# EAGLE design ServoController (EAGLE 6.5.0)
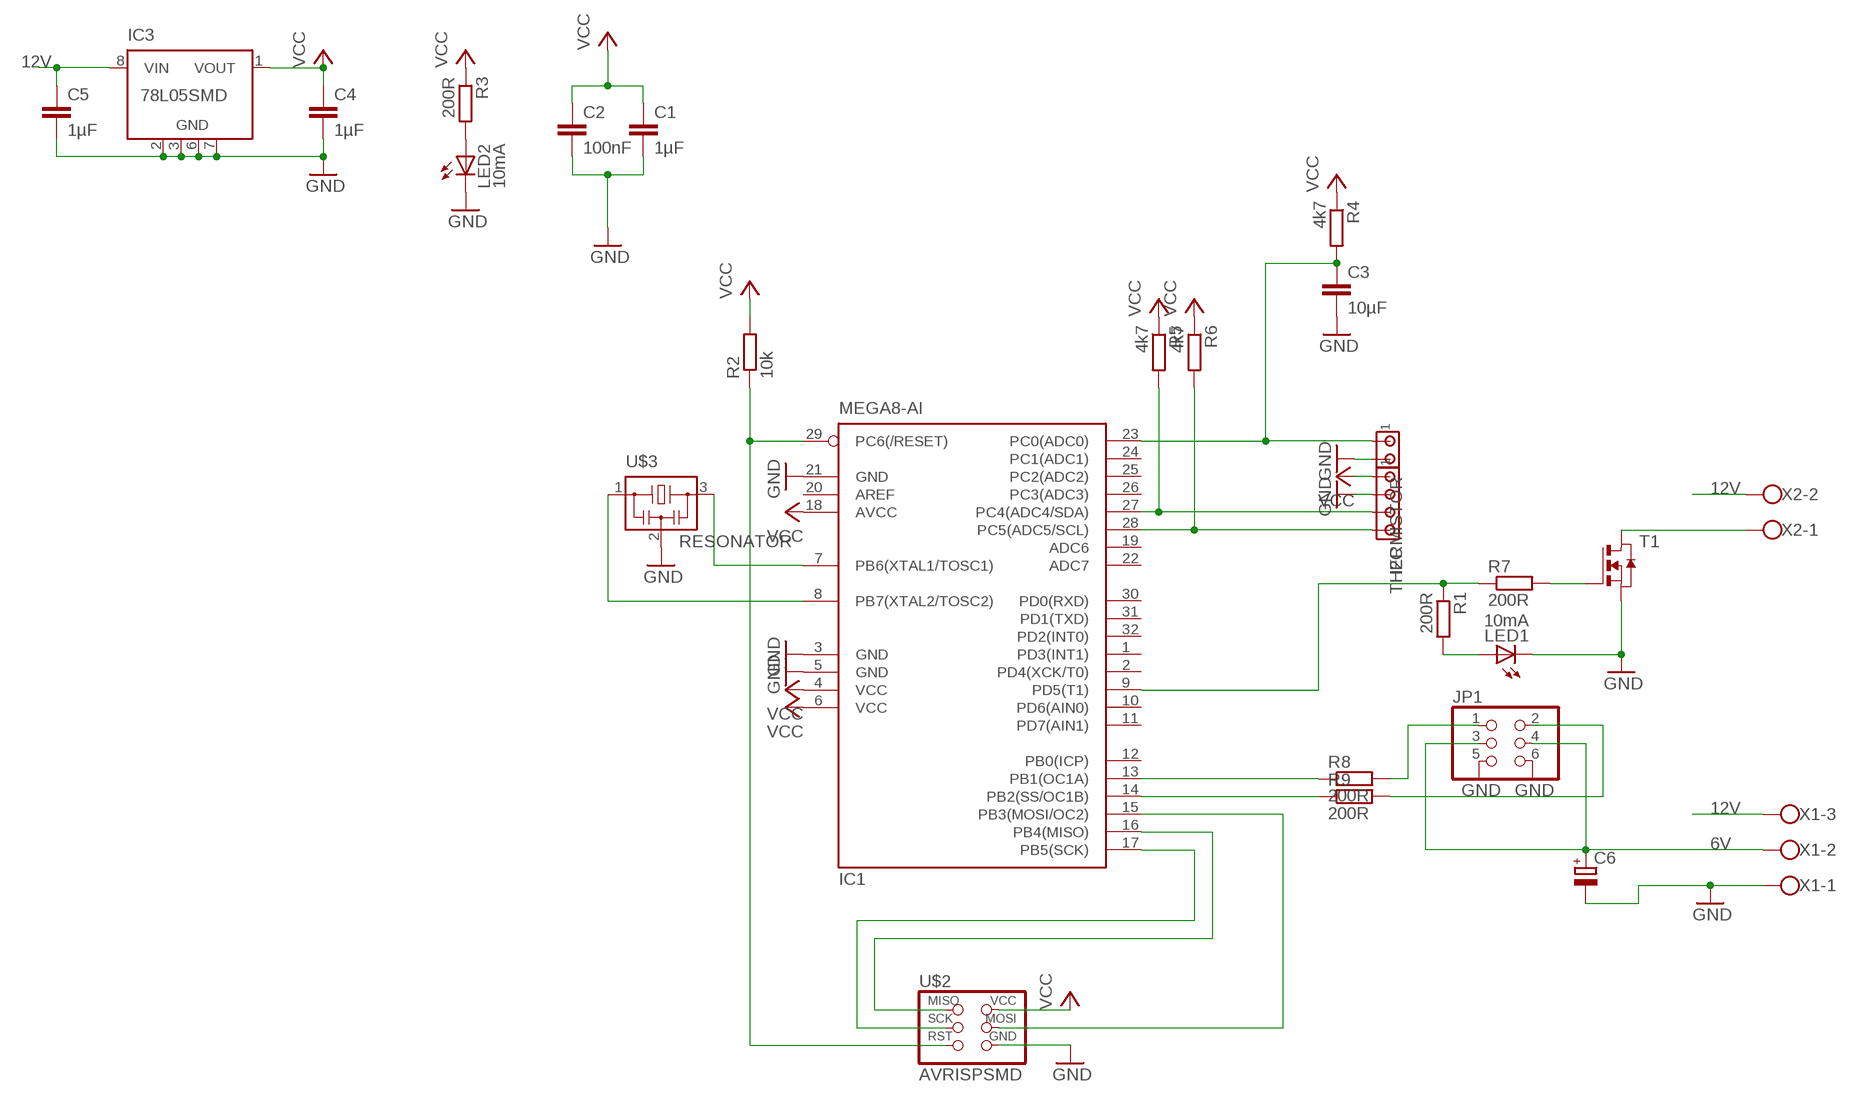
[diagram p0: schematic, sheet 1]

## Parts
C1  1µF  C-EUC1206  [C1206]
C2  100nF  C-EUC1206  [C1206]
C3  10µF  C-EUC1206  [C1206]
C4  1µF  C-EUC1206  [C1206]
C5  1µF  C-EUC1206  [C1206]
C6  CPOL-EUE10-25  [EB25D]
I2C  MTA04-100  [10X04MTA]
IC1  MEGA8-AI  [TQFP32-08]
IC3  78L05SMD  [SO08]
JP1  PINHD-2X3-SMD  [2X03SMD]
LED1  10mA  LEDCHIPLED_1206  [CHIPLED_1206]
LED2  10mA  LEDCHIPLED_1206  [CHIPLED_1206]
R1  200R  R-EU_R1206  [R1206]
R2  10k  R-EU_R1206  [R1206]
R3  200R  R-EU_R1206  [R1206]
R4  4k7  R-EU_R1206  [R1206]
R5  4k7  R-EU_R1206  [R1206]
R6  4k7  R-EU_R1206  [R1206]
R7  200R  R-EU_R1206  [R1206]
R8  200R  R-EU_R1206  [R1206]
R9  200R  R-EU_R1206  [R1206]
T1  NMOSSOT23-6  [SOT23-6]
THERMISTOR  MTA02-100  [10X02MTA]
U$2  AVRISPSMD  [2X03SMD]
U$3  RESONATOR  [EFOBM]
X1  W237-103  [W237-103]
X2  W237-102  [W237-102]

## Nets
6V: C6.+ JP1.3 JP1.4 X1.2
12V: C5.1 IC3.8(VIN) X1.3 X2.2
GND: C1.2 C2.2 C3.2 C4.2 C5.2 C6.- I2C.2 IC1.3(GND) IC1.5(GND) IC1.21(GND) IC3.2(GND) IC3.3(GND) IC3.6(GND) IC3.7(GND) JP1.5 JP1.6 LED1.C LED2.C T1.4(S) THERMISTOR.2 U$2.6(GND) U$3.2 X1.1
N$1: IC1.13(PB1(OC1A)) R8.1
N$2: IC1.29(PC6(/RESET)) R2.1 U$2.5(RST)
N$3: JP1.2 R9.2
N$4: IC1.15(PB3(MOSI/OC2)) U$2.4(MOSI)
N$5: IC1.16(PB4(MISO)) U$2.1(MISO)
N$6: IC1.8(PB7(XTAL2/TOSC2)) U$3.1
N$7: IC1.7(PB6(XTAL1/TOSC1)) U$3.3
N$8: IC1.17(PB5(SCK)) U$2.3(SCK)
N$9: IC1.9(PD5(T1)) R1.1 R7.1
N$10: LED1.A R1.2
N$11: T1.1(D) T1.2(D) T1.5(D) T1.6(D) X2.1
N$12: LED2.A R3.2
N$13: I2C.3 IC1.27(PC4(ADC4/SDA)) R5.2
N$14: I2C.4 IC1.28(PC5(ADC5/SCL)) R6.2
N$15: C3.1 IC1.23(PC0(ADC0)) R4.2 THERMISTOR.1
N$16: R7.2 T1.3(G)
N$17: IC1.14(PB2(SS/OC1B)) R9.1
N$18: JP1.1 R8.2
VCC: C1.1 C2.1 C4.1 I2C.1 IC1.4(VCC) IC1.6(VCC) IC1.18(AVCC) IC3.1(VOUT) R2.2 R3.1 R4.1 R5.1 R6.1 U$2.2(VCC)
Unconnected: IC1.1(PD3(INT1)) IC1.2(PD4(XCK/T0)) IC1.10(PD6(AIN0)) IC1.11(PD7(AIN1)) IC1.12(PB0(ICP)) IC1.19(ADC6) IC1.20(AREF) IC1.22(ADC7) IC1.24(PC1(ADC1)) IC1.25(PC2(ADC2)) IC1.26(PC3(ADC3)) IC1.30(PD0(RXD)) IC1.31(PD1(TXD)) IC1.32(PD2(INT0)) IC3.4(NC) IC3.5(NC)

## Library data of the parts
C1-C5 = resistor:C-EU: CAPACITOR, European symbol
C6 = rcl:CPOL-EU: POLARIZED CAPACITOR, European symbol
I2C = con-amp:MTA04-100: AMP connector
IC1 = atmel:MEGA8: MICROCONTROLLER 8 Kbytes FLASH, 1 kbytes SRAM, 512 bytes EEPROM, USART, 6-channel 10 bit ADC, 2-channel 8 bit ADC Pin compatible with Atmega48, ATMega88, ATMega168 Source: avr.lbr; MPN: ATMEGA8-16AU; OC_FARNELL: 9171371; OC_NEWARK: 73M8863
IC3 = linear:78L*SMD: Positive VOLTAGE REGULATOR
JP1 = fab:PINHD-2X3-SMD: PIN HEADER
LED1 LED2 = led:LED: LED
R1-R9 = resistor:R-EU_: RESISTOR, European symbol
T1 = zetex:NMOSSOT23-6: MOS FET; OC_FARNELL: unknown; OC_NEWARK: unknown
THERMISTOR = con-amp:MTA02-100: AMP connector
U$2 = fab:AVRISP
U$3 = fab:RESONATOR
X1 = con-wago-500:W237-103: WAGO SCREW CLAMP; MPN: 237-103; OC_FARNELL: unknown; OC_NEWARK: 18M7116
X2 = con-wago-500:W237-102: WAGO SCREW CLAMP; MPN: 237-102; OC_FARNELL: unknown; OC_NEWARK: 70K9898

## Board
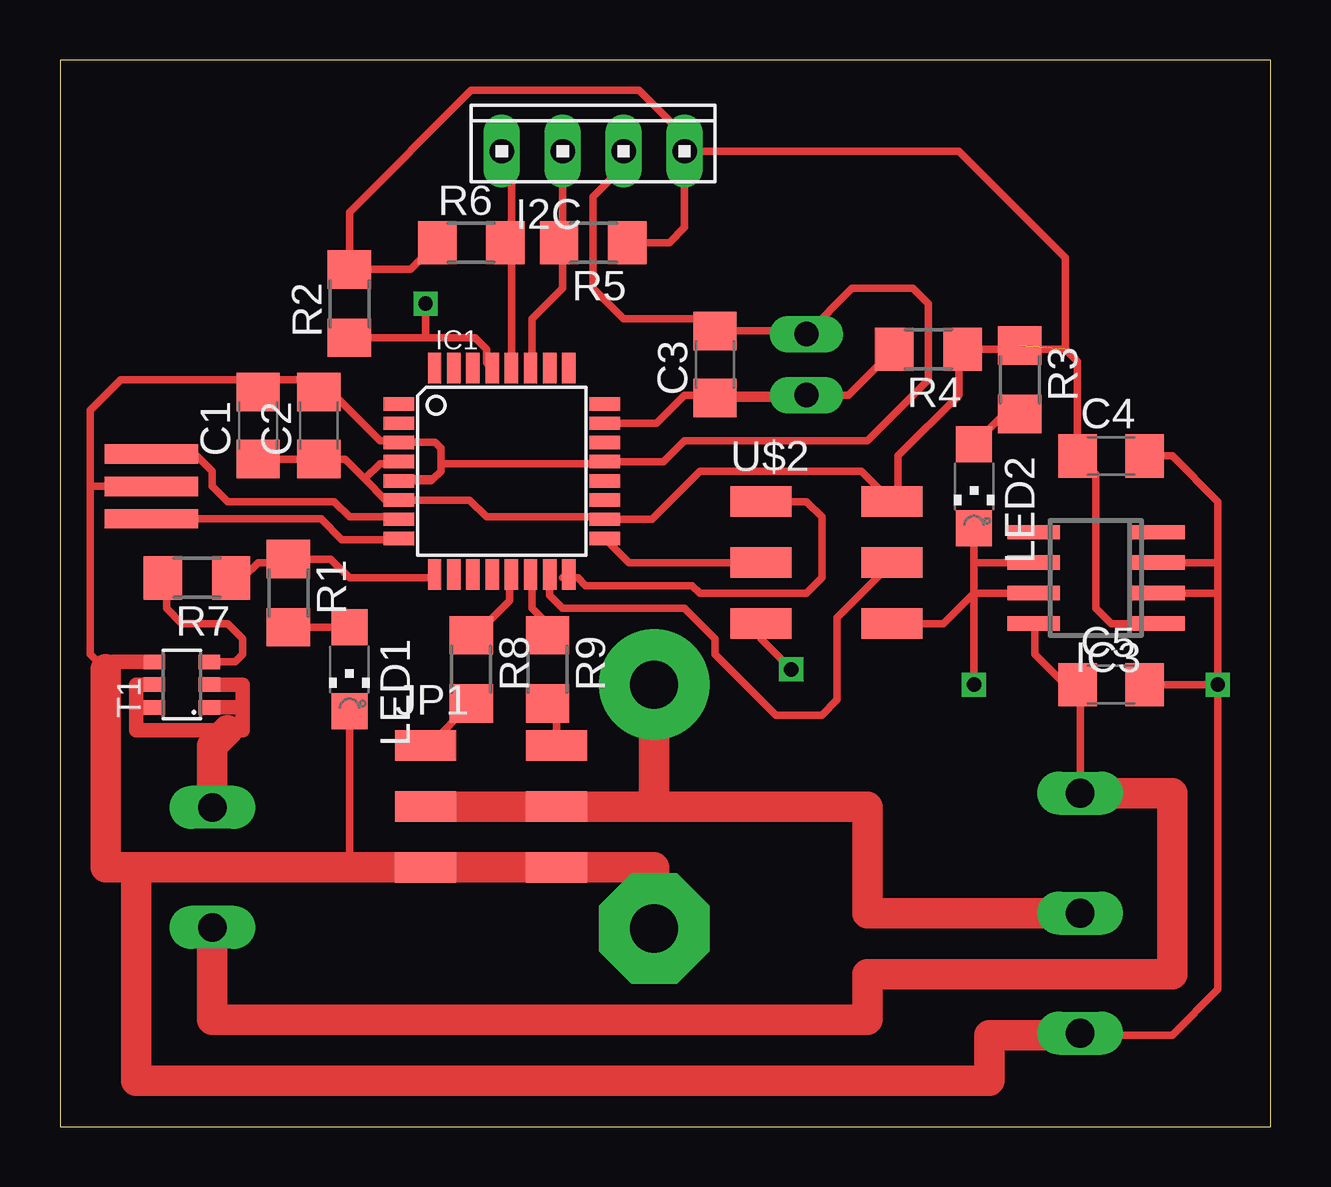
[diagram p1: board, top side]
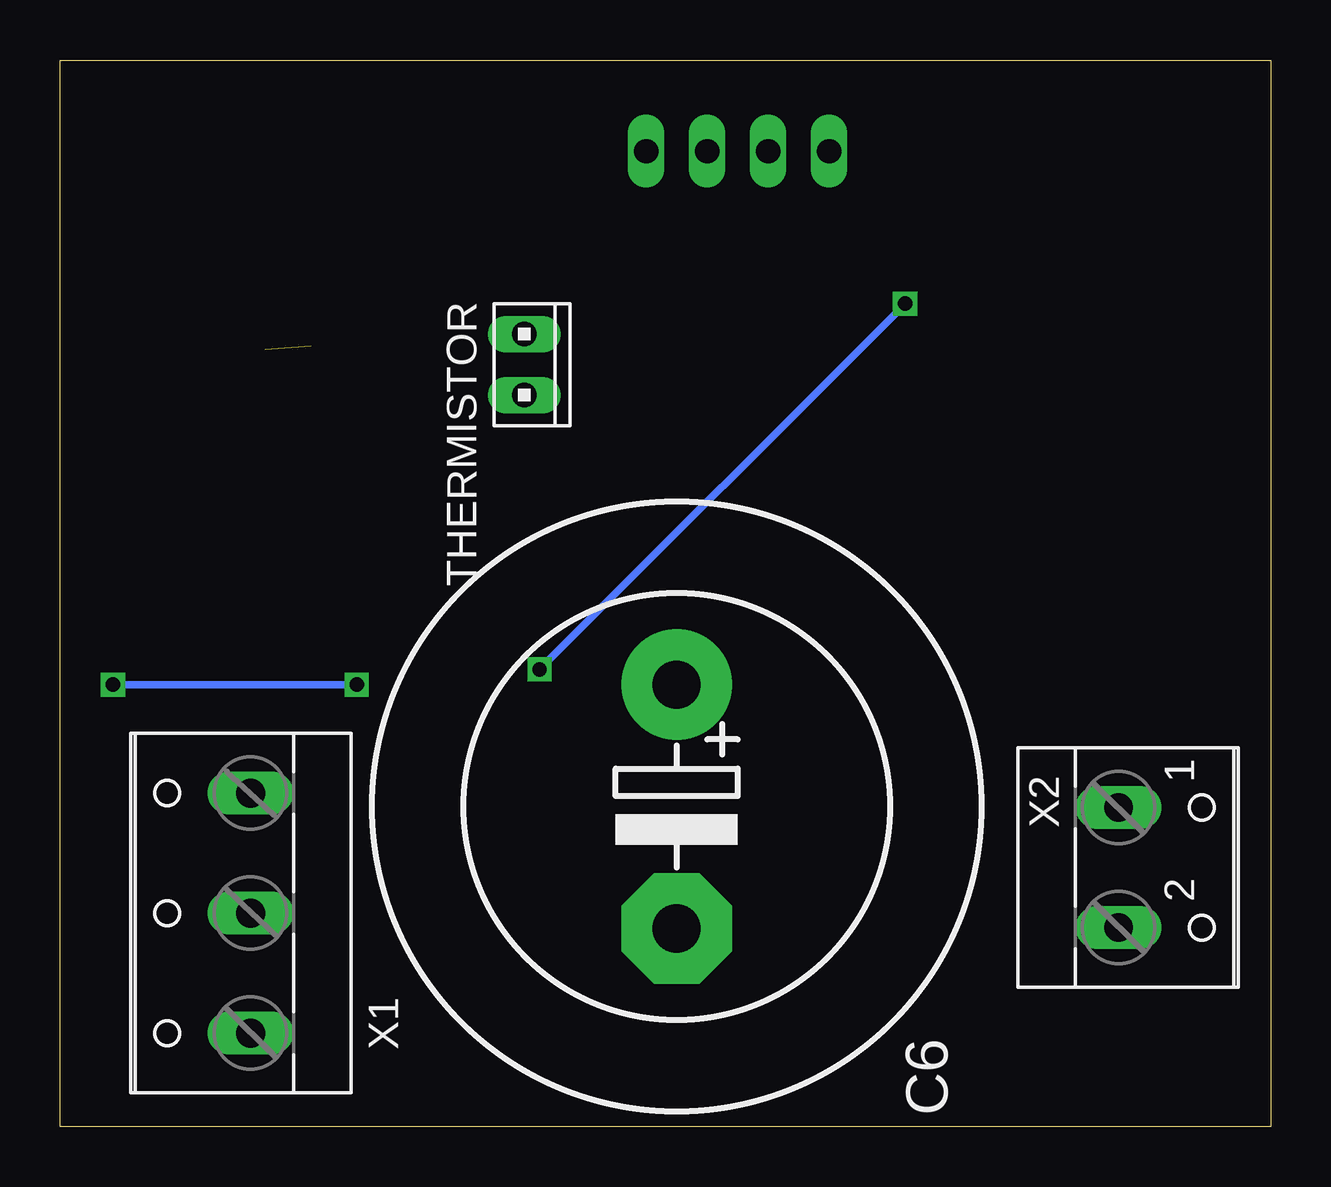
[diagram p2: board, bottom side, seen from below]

Size 50.47 x 44.44 mm. Coordinates in mm from the lower left corner, seen from the top.
Outline: 0,0 50.47,0 50.47,44.44 0,44.44 0,0
Copper layers (1*16): Top 0.035mm / dielectric 1.5mm / Bottom 0.035mm
Design rules "fab": minimum track width 0.3mm, minimum drill 32mil, track to track 0.315mm, track to pad 0.315mm, pad to pad 0.315mm, via to via 0.315mm, smd to smd 0.315mm, copper to edge 40mil, drill to drill 16mil, minimum pad ring 10mil, minimum via ring 8mil, stop-mask expansion 4mil, vias tented up to drill 0mil, thermal gap 10mil

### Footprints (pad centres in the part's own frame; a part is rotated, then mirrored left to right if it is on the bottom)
C1206 = smd 1.6 x 1.8: 1 -1.4,0; 2 1.4,0
EB25D = drill 2.007 pad 4.597: + -5.08,0 | drill 2.007 pad 4.597 octagon: - 5.08,0
10X04MTA = drill 1.016 long: 1 3.81,0; 2 1.27,0; 3 -1.27,0; 4 -3.81,0
TQFP32-08 = smd 1.27 x 0.559: 1 -4.293,2.8; 2 -4.293,2; 3 -4.293,1.2; 4 -4.293,0.4; 5 -4.293,-0.4; 6 -4.293,-1.2; 7 -4.293,-2; 8 -4.293,-2.8; 17 4.293,-2.8; 18 4.293,-2; 19 4.293,-1.2; 20 4.293,-0.4; 21 4.293,0.4; 22 4.293,1.2; 23 4.293,2; 24 4.293,2.8 | smd 0.559 x 1.27: 9 -2.8,-4.293; 10 -2,-4.293; 11 -1.2,-4.293; 12 -0.4,-4.293; 13 0.4,-4.293; 14 1.2,-4.293; 15 2,-4.293; 16 2.8,-4.293; 25 2.8,4.293; 26 2,4.293; 27 1.2,4.293; 28 0.4,4.293; 29 -0.4,4.293; 30 -1.2,4.293; 31 -2,4.293; 32 -2.8,4.293
SO08 = smd 0.6 x 2.2: 1 -1.905,-2.6; 2 -0.635,-2.6; 3 0.635,-2.6; 4 1.905,-2.6; 5 1.905,2.6; 6 0.635,2.6; 7 -0.635,2.6; 8 -1.905,2.6
2X03SMD = smd 2.54 x 1.27: 1 -2.54,2.54; 2 2.92,2.54; 3 -2.54,0; 4 2.92,0; 5 -2.54,-2.54; 6 2.92,-2.54
CHIPLED_1206 = smd 1.5 x 1.5: A 0,-1.75; C 0,1.75
R1206 = smd 1.6 x 1.803: 1 -1.422,0; 2 1.422,0
SOT23-6 = smd 0.6 x 0.9: 1 -0.95,-1.15; 2 0,-1.15; 3 0.95,-1.15; 4 0.95,1.15; 5 0,1.15; 6 -0.95,1.15
10X02MTA = drill 1.016 long: 1 1.27,0; 2 -1.27,0
EFOBM = smd 0.8 x 3.9: 1 -1.35,0; 2 0,0; 3 1.35,0
W237-103 = drill 1.194 long: 1 -5,-1.29; 2 0,-1.29; 3 5,-1.29
W237-102 = drill 1.194 long: 1 -2.5,-1.27; 2 2.5,-1.27

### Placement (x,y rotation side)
C1  8.26,29.21 90 top
C2  10.79,29.21 90 top
C3  27.3,31.75 90 top
C4  43.81,27.94 0 top
C5  43.81,18.41 0 top
C6  24.77,13.34 270 bottom
I2C  22.23,40.64 0 top
IC1  18.41,27.3 0 top
IC3  43.18,22.86 90 top
JP1  17.78,13.34 0 top
LED1  12.06,19.05 180 top
LED2  38.1,26.67 180 top
R1  9.53,22.23 270 top
R2  12.06,34.29 90 top
R3  40.01,31.11 270 top
R4  36.2,32.38 180 top
R5  22.23,36.83 180 top
R6  17.14,36.83 0 top
R7  5.71,22.86 180 top
R8  17.14,19.05 270 top
R9  20.32,19.05 270 top
T1  5.08,18.41 90 top
THERMISTOR  31.11,31.75 270 bottom
U$2  31.75,23.5 0 top
U$3  3.81,26.67 90 top
X1  43.81,8.89 90 bottom
X2  5.08,10.79 270 bottom

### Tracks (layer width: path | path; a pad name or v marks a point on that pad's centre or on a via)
6V
  Top 1.27: JP1.3 JP1.4 24.77,13.34 | 24.77,13.34 33.66,13.34 33.66,8.89 X1.2 | 24.77,13.34 C6.+
12V
  Top 0.305: X1.3 42.52,18.3 C5.1 41.91,18.41 40.64,19.68 40.64,20.89 IC3.8
  Top 1.27: X1.3 46.35,13.89 46.35,6.35 33.66,6.35 33.66,4.45 6.35,4.45 X2.2
GND  (via drill 0.6)
  Top 0.305: 8.26,31.11 10.79,31.11 | 10.79,31.11 13.34,28.57 14.05,28.57 IC1.3 15.63,28.5 15.88,28.26 15.88,27.62 | 15.56,26.99 15.88,27.3 15.88,27.62 | 15.56,26.99 14.21,26.99 IC1.5 15.47,26.91 15.56,26.99 | 15.88,27.62 22.62,27.62 IC1.21 25.16,27.7 26.04,28.57 33.66,28.57 36.2,31.11 36.2,34.29 35.56,34.92 33.02,34.92 THERMISTOR.2 30.98,33.15 C3.2 26.8,33.66 23.5,33.66 22.23,34.92 22.23,38.73 23.5,40.01 I2C.2 23.5,41.91 | LED1.C 12.06,10.79 | v48.26,18.41 48.26,5.71 46.35,3.81 42.6,3.81 X1.1 | 46.35,18.41 C5.2 v48.26,18.41 | 38.1,22.23 36.83,20.95 U$2.6 | IC3.7 38.1,22.23 | IC3.3 48.26,23.5 | 48.26,23.5 48.26,22.23 | 48.26,22.23 IC3.2 | 38.73,23.5 IC3.6 38.1,23.5 | C4.2 46.35,27.94 48.26,26.04 48.26,23.5 | C2.2 10.79,31.11 | C1.2 8.26,31.11 | 8.26,31.11 2.54,31.11 1.27,29.84 1.27,26.67 | 1.27,26.67 1.27,19.68 1.91,19.05 | U$3.2 1.27,26.67 | LED2.C 38.1,23.5 | 38.1,23.5 38.1,22.23 | 38.1,22.23 v38.1,18.41 | v48.26,18.41 48.26,22.23
  Top 0.61: T1.4 2.22,19.36 1.91,19.05
  Top 1.27: 3.17,10.79 12.06,10.79 JP1.5 JP1.6 24.77,10.79 C6.- | 3.17,10.79 3.17,1.91 38.73,1.91 38.73,3.81 42.52,3.81 X1.1 | 1.91,19.05 1.91,10.79 3.17,10.79
  Bottom 0.305: v38.1,18.41 v48.26,18.41
N$1
  Top 0.305: R8.1 17.78,20.95 18.73,21.91 18.73,22.93 IC1.13
N$2  (via drill 0.6)
  Top 0.305: R2.1 15.24,32.87 | 15.24,32.87 17.3,32.87 17.78,32.38 17.78,31.83 IC1.29 | U$2.5 29.21,20.32 v30.48,19.05 | v15.24,34.29 15.24,32.87
  Bottom 0.305: v15.24,34.29 v30.48,19.05
N$3
  Top 0.305: JP1.2 20.7,17.25 R9.2
N$4
  Top 0.305: IC1.15 20.41,22.13 20.95,21.59 26.04,21.59 27.3,20.32 27.3,19.68 29.84,17.14 31.75,17.14 32.38,17.78 32.38,21.21 U$2.4 33.66,23.5
N$5
  Top 0.305: IC1.16 21.11,23.01 20.95,22.86 21.59,22.86 21.91,22.54 26.35,22.54 26.67,22.23 31.11,22.23 31.75,22.86 31.75,25.4 31.11,26.04 U$2.1
N$6
  Top 0.305: U$3.1 10.88,25.32 11.75,24.45 14.06,24.45 IC1.8
N$7
  Top 0.305: U$3.3 5.63,28.02 6.35,27.3 6.35,26.67 6.99,26.04 11.43,26.04 12.06,25.4 14.03,25.4 IC1.7
N$8
  Top 0.305: U$2.3 23.72,23.5 IC1.17
N$9
  Top 0.305: IC1.9 15.46,22.86 12.06,22.86 11.28,23.65 R1.1 9.37,23.5 8.26,23.5 7.62,22.86 R7.1
N$10
  Top 0.305: LED1.A R1.2
N$11
  Top 0.61: T1.2 7.62,18.41 7.62,17.46 | T1.5 3.17,18.41 3.17,17.46 | 3.17,17.46 T1.6 | T1.1 7.62,17.46 | 3.17,17.46 3.17,16.51 6.99,16.51 7.62,16.51 7.62,17.46
  Top 1.27: X2.1 6.35,15.88 6.99,16.51
N$12
  Top 0.305: R3.2 39.37,29.69 LED2.A
N$13
  Top 0.305: IC1.27 19.61,31.68 19.68,31.75 19.68,33.66 20.95,34.92 20.95,36.83 | 20.95,36.83 I2C.3 | R5.2 20.95,36.83
N$14
  Top 0.305: IC1.28 18.82,36.83 | 18.82,36.83 18.82,40.24 I2C.4 | R6.2 18.82,36.83
N$15
  Top 0.305: IC1.23 24.86,29.3 26.04,30.48 THERMISTOR.1 | THERMISTOR.1 32.87,30.48 R4.2 | C3.1 30.98,30.35 THERMISTOR.1
N$16
  Top 0.305: T1.3 7.3,19.36 7.62,19.68 7.62,20.32 6.99,20.95 5.08,20.95 4.45,21.59 4.45,23.34 R7.2
N$17
  Top 0.305: R9.1 20.32,20.95 19.68,21.59 19.68,22.94 IC1.14
N$18
  Top 0.305: JP1.1 15.39,15.88 R8.2
VCC  (1 unrouted)
  Top 0.305: 12.7,26.99 13.58,26.11 IC1.6 17.07,26.11 17.78,25.4 22.61,25.4 IC1.18 24.67,25.3 26.67,27.3 33.4,27.3 U$2.2 34.92,26.29 34.92,27.94 37.47,30.48 37.47,32.23 R4.1 | 12.7,26.99 13.34,27.62 14.04,27.62 IC1.4 | IC3.1 43.81,20.95 43.18,21.59 43.18,27.18 C4.1 42.41,31.88 41.91,32.38 | 41.91,32.38 R4.1 | R4.1 37.62,31.9 | C1.1 C2.1 11.88,27.81 12.7,26.99 | 41.91,32.38 41.91,36.2 37.47,40.64 I2C.1 | R5.1 25.4,36.83 26.04,37.47 I2C.1 | R6.1 14.61,35.71 R2.2 12.06,38.1 17.14,43.18 24.13,43.18 26.04,41.27 I2C.1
